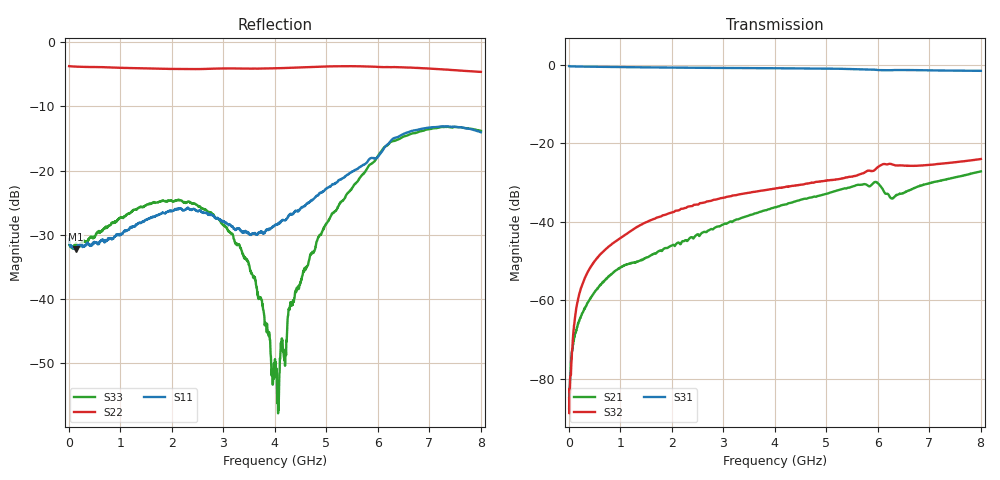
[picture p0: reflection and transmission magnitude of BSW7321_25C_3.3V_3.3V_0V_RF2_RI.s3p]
! Product: BSW7321
! Temp: 25C
! VDD: 3.300
! Control_Hi: 3.300
! Control_Lo: 0.000
! Logic State: RF2
! Port 1: RFC
! Port 2: RF1
! Port 3: RF2
! V1 = 0.00
! V2 = 0.00
! V3 = 0.00
! V4 = 0.00
# Hz S  RI  R 50
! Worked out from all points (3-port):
!   1601 points, 5 MHz to 8.005 GHz, reference 50 ohm
!   strongest paths, dB at 5 MHz, 2.005 GHz, 4.005 GHz, 6.005 GHz, 8.005 GHz:
!     S31: -0.4, -0.7, -0.9, -1.4, -1.6
!     S32: -85.0, -37.6, -31.6, -26.1, -24.0
!     S21: -87.5, -46.1, -36.3, -30.2, -27.2
!   lowest |S11| = -32.3 dB at 135 MHz (marker M1), VSWR 1.05, Z = 52.4 - j0.731 ohm
!   |S11| at or under -10 dB: start of sweep to end of sweep
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5000000  0.0292 -0.00393  1.39e-05 -2.35e-05  0.9564 -0.0123
         1.02e-05 -4.07e-05  -0.6492 0.00647  3.63e-05 1.07e-05
         0.9565 -0.0121  2.21e-05 5.2e-05  0.0284 -0.00307
1.35e8  0.0233 -0.00697  -0.000388 0.000119  0.9237 -0.2114
        -0.000361 0.000141  -0.6293 0.1409  -6.47e-05 0.000702
        0.9238 -0.2114  -8.63e-05 0.000714  0.0259 -0.0074
1.005e9  -0.0249 -0.0193  0.00244 0.000934  -0.0569 -0.9302
         0.00245 0.000918  0.0132 0.631  0.00613 0.0009
         -0.0569 -0.9305  0.00614 0.000917  -0.0253 -0.0352
1.935e9  -0.00649 0.0475  0.00276 -0.00382  -0.918 -0.0143
         0.00278 -0.00381  0.6169 0.0506  0.00389 -0.0121
         -0.9181 -0.0145  0.00389 -0.0121  -0.0389 0.043
2.95e9  0.0405 0.00573  -0.00624 -0.0063  0.0363 0.9074
        -0.00625 -0.0063  0.00221 -0.6231  -0.0187 -0.00669
        0.0362 0.9074  -0.0187 -0.00669  0.0312 0.025
4.005e9  0.0299 -0.0227  -0.0101 0.0115  0.8881 -0.1462
         -0.0101 0.0115  -0.6168 0.101  -0.00856 0.0249
         0.8884 -0.1463  -0.00857 0.0249  -0.00126 -0.00316
4.91e9  -0.036 -0.0576  0.0146 0.0162  -0.0428 -0.8892
        0.0146 0.0161  -0.0159 0.6447  0.0273 0.0182
        -0.0427 -0.8891  0.0272 0.0182  -0.0203 0.0255
5.84e9  -0.0745 0.0978  0.0184 -0.0213  -0.8668 -0.0155
        0.0183 -0.0213  0.6261 0.1566  0.0333 -0.03
        -0.8665 -0.0155  0.0333 -0.0299  0.0323 0.1057
6.875e9  0.2065 0.049  -0.0175 -0.0234  0.0533 0.8475
         -0.0176 -0.0235  0.1784 -0.6002  -0.0408 -0.0325
         0.0535 0.8477  -0.0407 -0.0324  0.1975 -0.05
8.005e9  -0.0497 -0.1922  -0.0274 0.0342  0.7931 -0.2586
         -0.0273 0.0341  -0.5863 -0.0132  -0.0345 0.0526
         0.793 -0.2585  -0.0345 0.0525  -0.051 -0.1973
